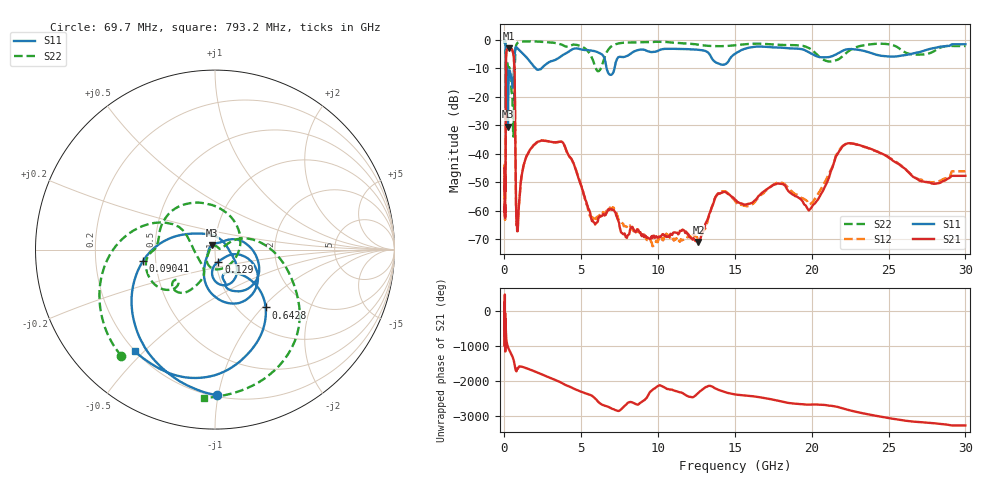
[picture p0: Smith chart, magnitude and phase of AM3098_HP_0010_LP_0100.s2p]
! Date/Time: Thu, Feb 28, 2019 8:32 AM
! Network Analyzer: Agilent Technologies E8364B Rev: A.07.50.67
! Sweep from 0.010 to 30.000 GHz, 1601 Points, Sweep Type: LOG
! Power Supply: 5.022 V, 0.002 A
# Hz S DB R 50
!freq MagS11 AngS11 MagS21 AngS21 MagS12 AngS12 MagS22 AngS22
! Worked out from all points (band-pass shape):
!   1601 points, 10 MHz to 30 GHz, reference 50 ohm
!   highest |S21| = -3.03 dB at 266.5 MHz (marker M1); lowest = -70.9 dB at 12.62 GHz (marker M2)
!   |S21| within 3 dB of the highest: 106.2 MHz to 601.5 MHz (495.3 MHz wide, 140 % of centre)
!   lowest |S11| = -30.5 dB at 228.2 MHz (marker M3), VSWR 1.06, Z = 48.3 + j2.37 ohm
!   |S11| at or under -10 dB: 176.3 MHz to 619.1 MHz (442.8 MHz wide, 111 % of centre); 2.012 GHz to 2.429 GHz (417 MHz wide, 18.8 % of centre); 6.645 GHz to 7.166 GHz (521.1 MHz wide, 7.55 % of centre)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
!   |S22| runs from -34.0 to -0.5 dB; largest |S21 - S12| = 0.0087
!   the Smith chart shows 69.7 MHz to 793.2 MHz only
!   S11 on the Smith chart (normalised r, x): 69.7 MHz: 0.21, -0.99; 90.41 MHz: 0.43, -0.06; 129 MHz: 1.03, -0.14; 642.8 MHz: 1.32, -1.04; 793.2 MHz: 0.20, -0.47
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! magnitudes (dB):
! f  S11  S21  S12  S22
! 10 MHz  -0.3  -44.9  -45.3  -0.5
! 38.04 MHz  -0.5  -58.3  -62.3  -0.8
! 69.7 MHz  -1.8  -51.2  -51.1  -2.0
! 90.41 MHz  -7.9  -19.5  -19.6  -9.3
! 99.92 MHz  -23.8  -8.0  -8.0  -17.4
! 129 MHz  -23.2  -4.1  -4.0  -11.1
! 144.7 MHz  -13.8  -3.6  -3.6  -10.2
! 185.8 MHz  -11.2  -3.5  -3.5  -8.1
! 228.2 MHz  -30.5  -3.1  -3.1  -9.6
! 266.5 MHz  -14.7  -3.0  -3.0  -9.9
! 550.5 MHz  -16.8  -4.4  -4.3  -30.0
! 642.8 MHz  -7.4  -9.8  -9.7  -16.4
! 793.2 MHz  -2.8  -64.1  -63.6  -1.6
! 2.084 GHz  -10.4  -36.1  -36.2  -0.7
! 3.798 GHz  -5.5  -36.1  -36.1  -2.0
! 5.697 GHz  -3.9  -63.6  -62.1  -6.5
! 7.926 GHz  -5.9  -69.3  -65.6  -1.1
! 12.62 GHz  -3.6  -70.9  -69.2  -1.8
! 14.16 GHz  -8.8  -53.6  -53.2  -2.3
! 20 GHz  -5.0  -58.6  -57.2  -3.6
! 22.67 GHz  -3.4  -36.4  -36.5  -3.2
! 30 GHz  -1.7  -47.8  -46.2  -2.3
